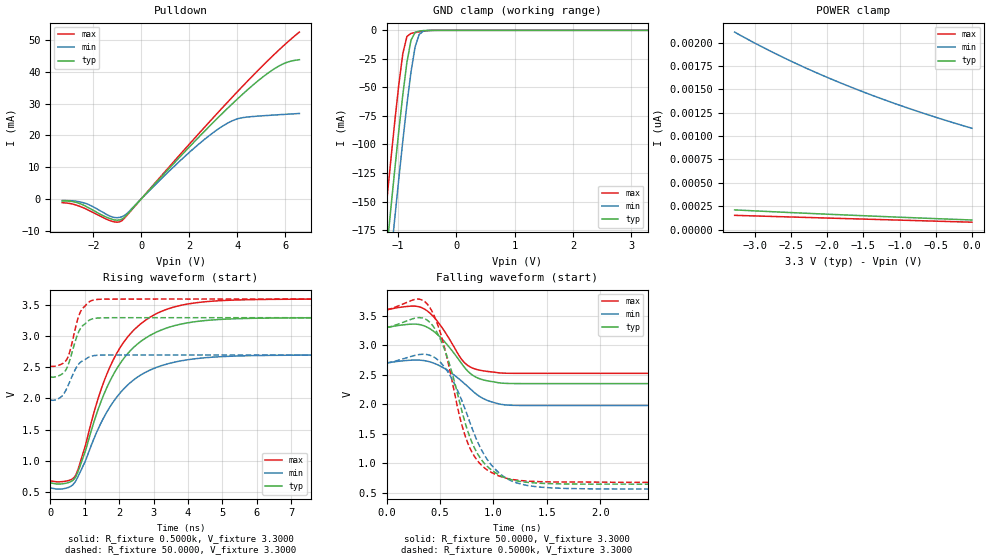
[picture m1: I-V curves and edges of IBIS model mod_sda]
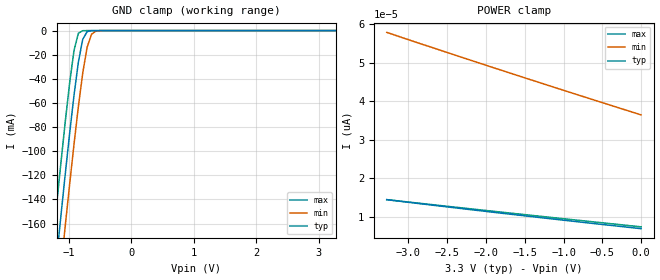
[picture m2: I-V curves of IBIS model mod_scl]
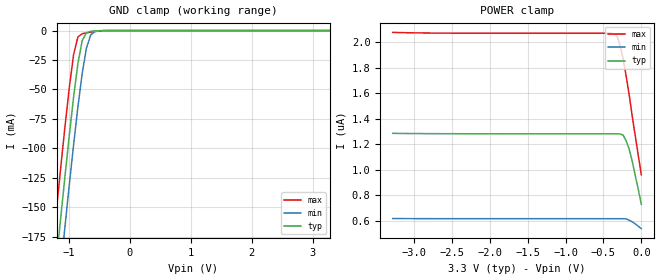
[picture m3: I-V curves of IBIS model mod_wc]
| IBIS (I/O, Buffer, Information, Specification) Model, officially
| electronic behavioral standard for Buffer structures of digital pins.
[IBIS ver]  4.0
[File name] m24c08_fb2_tssop8.ibs
[File Rev]  1.0
[Date]   23 Oct 2014
[Source]   CAD & Design Services (Catania) - STMicroelectronics
[Notes]
   (Note1)  This IBIS model includes the TSSOP8 package data
   (Note2)  This IBIS model has some Notes about the non-monotonicity
   of the I-V curves, but they are not indicative of problems
   inside the model;
[Copyright] (c) 2014 STMicroelectronics
|   Component M24C08
[Component] M24C08
[Manufacturer] STMicroelectronics
[Package]
| variable   typ   min   max
R_pkg   0.0   0.0   0.0
L_pkg   0.0H   0.0H   0.0H
C_pkg   0.0F   0.0F   0.0F
[Pin]  signal_name   model_name   R_pin   L_pin   C_pin
1   1NC   NC   NA   NA   NA
2   2NC   NC   NA   NA   NA
3   3NC   NC   NA   NA   NA
4   VSS   GND   NA   NA   NA
5   SDA   mod_sda   NA   NA   NA
6   SCL   mod_scl   NA   NA   NA
7   WCN   mod_wc   NA   NA   NA
8   VCC   POWER   NA   NA   NA
[Package Model]  182696_TSSOP8
[Define Package Model]  182696_TSSOP8
[Manufacturer]  STMicroelectronics
[OEM]  STMicroelectronics
[Description]  8 pin TSSOP package
[Number Of Pins]  8
[Pin Numbers]
|Pin Num   Terminal Name
1   | net1
2   | net2
3   | net3
4   | net4_GND
5   | net5
6   | net6
7   | net7
8   | net8_VDD
[Model Data]
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[End Model Data]
[End Package Model]
| Models and submodels in the file (3): mod_sda (I/O_open_drain), mod_scl (Input), mod_wc (Input)
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|   Model mod_sda
[Model]   mod_sda
Model_type I/O_open_drain
Polarity   Non-Inverting
Vinl   =   1.000V
Vinh   =   2.300V
Vmeas  =   1.650V
Cref   =   10pF
Rref   =   1k
Vref   =   3.300V
C_comp   2.024pF   1.846pF   2.119pF
[Temperature Range]  25.0000   85.0000   -40.0000
[Voltage Range]   3.3000V   2.7000V   3.6000V
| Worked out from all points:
|   slope of the pulldown table from 0 to 0.495 V, typ, clamps not added: 120 ohm
|   GND clamp passes 1 mA (typ) near -0.66 V on its own axis
|   rising waveform, R_fixture 0.5000k, V_fixture 3.3000: 20-80 % time 1.3ns typ, 1.35ns min, 1.26ns max; typ from 0.641 V to 3.3 V
|   rising waveform, R_fixture 50.0000, V_fixture 3.3000: 20-80 % time 341ps typ, 385ps min, 311ps max; typ from 2.35 V to 3.3 V
|   falling waveform, R_fixture 50.0000, V_fixture 3.3000: 20-80 % time 256ps typ, 294ps min, 229ps max; typ from 3.3 V to 2.35 V
|   falling waveform, R_fixture 0.5000k, V_fixture 3.3000: 20-80 % time 275ps typ, 318ps min, 246ps max; typ from 3.3 V to 0.641 V
[Pulldown]
|Voltage   I(typ)   I(min)   I(max)
-3.3V     -676uA     -510uA     -1.207mA
-2.8V     -934uA     -640uA     -1.752mA
-2.3V     -2.374mA   -1.459mA   -3.192mA
-1.3V     -6.204mA   -5.444mA   -6.872mA
-1V       -6.712mA   -5.933mA   -7.342mA
-800mV    -6.356mA   -5.606mA   -6.844mA
2V        16.3mA     14.61mA    17.19mA
3.5V      27.8mA     23.42mA    29.64mA
4.2V      32.78mA    25.56mA    35.26mA
5.4V      40.23mA    26.36mA    44.43mA
6V        42.81mA    26.65mA    48.69mA
6.6V      43.87mA    26.91mA    52.57mA
[GND_clamp]
|Voltage   I(typ)   I(min)   I(max)
-3.3V     -1.349A    -1.389A    -1.31A
-1.27V    -231.2mA   -274.4mA   -188.5mA
-1.2V     -194.4mA   -237.6mA   -151.7mA
-1.13V    -158.2mA   -201.3mA   -115.6mA
-1.06V    -122.8mA   -165.5mA   -80.71mA
-920mV    -56.25mA   -96.78mA   -20.32mA
-850mV    -28.07mA   -64.93mA   -5.417mA
-780mV    -8.653mA   -36.52mA   -2.698mA
-710mV    -1.808mA   -14.73mA   -1.965mA
-640mV    -572.4uA   -3.659mA   -1.349mA
-570mV    -239.3uA   -797.2uA   -774.2uA
3.28V     102.3pA    1.222nA    72.37pA
[POWER_clamp]
|Voltage   I(typ)   I(min)   I(max)
-3.28V    211pA      2.113nA    152.6pA
-2.92V    197.4pA    1.962nA    144.5pA
-2.56V    184.4pA    1.824nA    136.4pA
-2.2V     171.8pA    1.696nA    128.3pA
-1.76V    157pA      1.552nA    118.5pA
-1.36V    144.1pA    1.431nA    109.6pA
-920mV    130.3pA    1.309nA    99.83pA
-480mV    117pA      1.197nA    90.07pA
0V        102.9pA    1.084nA    79.45pA
[Ramp]
| variable   typ   min   max
dV/dt_r   0.5713/0.4051n   0.4337/0.4647n   0.6471/0.3730n
dV/dt_f   0.5713/0.2890n   0.4337/0.3425n   0.6471/0.2608n
R_load = 50.0000
[Rising Waveform]
R_fixture= 0.5000k
V_fixture= 3.3000
V_fixture_min= 2.7000
V_fixture_max= 3.6000
|time   V(typ)   V(min)   V(max)
0s        641.5mV    561.3mV    674.3mV
470ps     638.1mV    558.4mV    671.6mV
730ps     731.3mV    664.8mV    756.9mV
1.01ns    1.139V     983.2mV    1.224V
1.43ns    1.886V     1.557V     2.069V
1.83ns    2.383V     1.946V     2.621V
2.35ns    2.783V     2.267V     3.056V
3.07ns    3.065V     2.498V     3.362V
4.87ns    3.27V      2.671V     3.572V
10ns      3.3V       2.7V       3.6V
[Rising Waveform]
R_fixture= 50.0000
V_fixture= 3.3000
V_fixture_min= 2.7000
V_fixture_max= 3.6000
|time   V(typ)   V(min)   V(max)
0s        2.348V     1.977V     2.522V
270ps     2.371V     2.008V     2.54V
370ps     2.405V     2.058V     2.567V
470ps     2.477V     2.151V     2.62V
570ps     2.625V     2.276V     2.76V
770ps     2.996V     2.51V      3.222V
870ps     3.12V      2.58V      3.386V
1.09ns    3.243V     2.656V     3.537V
1.27ns    3.287V     2.69V      3.586V
10ns      3.3V       2.7V       3.6V
[Falling Waveform]
R_fixture= 50.0000
V_fixture= 3.3000
V_fixture_min= 2.7000
V_fixture_max= 3.6000
|time   V(typ)   V(min)   V(max)
0s        3.3V       2.7V       3.6V
240ps     3.355V     2.745V     3.66V
340ps     3.333V     2.74V      3.624V
420ps     3.26V      2.708V     3.517V
500ps     3.139V     2.647V     3.345V
680ps     2.743V     2.423V     2.817V
740ps     2.598V     2.33V      2.684V
860ps     2.438V     2.143V     2.58V
1.08ns    2.356V     1.995V     2.527V
10ns      2.348V     1.977V     2.522V
[Falling Waveform]
R_fixture= 0.5000k
V_fixture= 3.3000
V_fixture_min= 2.7000
V_fixture_max= 3.6000
|time   V(typ)   V(min)   V(max)
0s        3.3V       2.7V       3.6V
290ps     3.464V     2.835V     3.779V
400ps     3.393V     2.831V     3.65V
560ps     2.837V     2.582V     2.828V
700ps     1.916V     2.079V     1.675V
780ps     1.438V     1.689V     1.257V
960ps     917.4mV    1.017V     865.2mV
1.18ns    715.4mV    692.8mV    724.5mV
1.94ns    646.1mV    566.4mV    680.8mV
10ns      641.5mV    561.3mV    674.3mV
|   Model mod_scl
[Model]   mod_scl
Model_type Input
Vinl   =   1.000V
Vinh   =   2.300V
C_comp   1.845pF   1.683pF   1.932pF
[Temperature Range]  25.0000   85.0000   -40.0000
[Voltage Range]   3.3000V   2.7000V   3.6000V
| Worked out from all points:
|   GND clamp passes 1 mA (typ) near -0.71 V on its own axis
[GND_clamp]
|Voltage   I(typ)   I(min)   I(max)
-3.3V     -1.323A    -1.364A    -1.283A
-1.27V    -225.4mA   -268.8mA   -181.3mA
-1.2V     -189.3mA   -232.7mA   -145.2mA
-1.13V    -153.7mA   -197mA     -109.8mA
-1.06V    -118.9mA   -161.8mA   -75.51mA
-920mV    -53.64mA   -94.29mA   -16.44mA
-850mV    -26.06mA   -63.01mA   -2.183mA
-780mV    -7.218mA   -35.12mA   -106.6uA
-710mV    -894.4uA   -13.78mA   -4.426uA
-640mV    -77.79uA   -3.065mA   -182.3nA
-570mV    -6.449uA   -442.1uA   -7.506nA
3.28V     6.813pA    40.1pA     6.665pA
[POWER_clamp]
|Voltage   I(typ)   I(min)   I(max)
-3.28V    14.38pA    57.84pA    14.39pA
-2.52V    12.55pA    52.74pA    12.71pA
-1.72V    10.69pA    47.47pA    10.97pA
0V        6.856pA    36.42pA    7.331pA
|   Model mod_wc
[Model]   mod_wc
Model_type Input
Vinl   =   1.000V
Vinh   =   2.300V
C_comp   1.845pF   1.683pF   1.932pF
[Temperature Range]  25.0000   85.0000   -40.0000
[Voltage Range]   3.3000V   2.7000V   3.6000V
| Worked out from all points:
|   GND clamp passes 1 mA (typ) near -0.66 V on its own axis
[GND_clamp]
|Voltage   I(typ)   I(min)   I(max)
-3.3V     -1.349A    -1.389A    -1.31A
-1.27V    -231.2mA   -274.4mA   -188.5mA
-1.2V     -194.4mA   -237.6mA   -151.7mA
-1.13V    -158.2mA   -201.3mA   -115.6mA
-1.06V    -122.8mA   -165.5mA   -80.71mA
-920mV    -56.25mA   -96.78mA   -20.32mA
-850mV    -28.07mA   -64.93mA   -5.417mA
-780mV    -8.653mA   -36.52mA   -2.698mA
-710mV    -1.808mA   -14.73mA   -1.965mA
-640mV    -572.4uA   -3.659mA   -1.349mA
-570mV    -239.3uA   -797.2uA   -774.2uA
3.28V     102.3pA    1.222nA    72.37pA
[POWER_clamp]
|Voltage   I(typ)   I(min)   I(max)
-3.28V    1.285uA    617.9nA    2.075uA
-2.48V    1.282uA    616.9nA    2.069uA
-400mV    1.282uA    616.6nA    2.069uA
-360mV    1.282uA    616.6nA    2.063uA
-320mV    1.282uA    616.6nA    2.046uA
-280mV    1.28uA     616.6nA    1.973uA
-240mV    1.271uA    616.6nA    1.869uA
-200mV    1.226uA    614.7nA    1.732uA
-160mV    1.161uA    604.7nA    1.587uA
-120mV    1.068uA    592nA      1.419uA
0V        730nA      538.6nA    960nA
